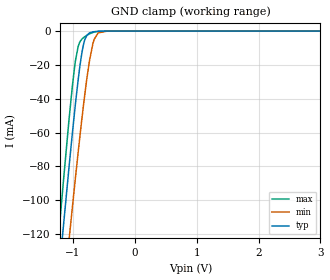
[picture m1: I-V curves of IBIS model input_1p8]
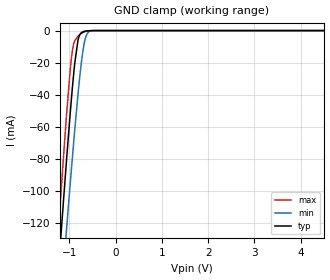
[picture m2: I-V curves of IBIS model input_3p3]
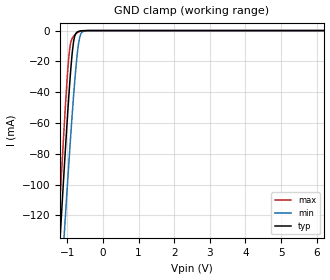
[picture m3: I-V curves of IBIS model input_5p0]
| Texas Instruments Incorporated
| ADS7028 Small, 8-Channel, 12-bit ADC with SPI Interface, GPIOs & CRC
[IBIS Ver]   4.1
[File name]   ads7028.ibs
[File Rev]   1.0
[Date]   03/21/2019
[Source]
| Texas Instruments Incorporated.
| Analog-eLab Design Center, HPA
| 12500 TI Blvd
| Dallas, TX -75243
[Notes]   Revision History:
| Rev 1.0: 03/21/2019
| - Initial version of the model
| - Model generated from simulations in SPECTRE
| - C_comp although listed in numerical order of value are
|   obtained from varying PVT conditions. For PVT conditions for
|   each specific value refer the buffer description under
|   respective [Model]. IBIS model user is responsible for using
|   appropriate C_comp to simulate for Signal Integrity.
| - Warnings regarding combined Non-monotonicity of various models have been
|   reviewd and considered minor and can be ignored.
| - Model names with a trailing _1p8 contain the model for 1.8V operation.
|   Model names with a trailing _2p5 contain the model for 2.5V operation.
|   Model names with a trailing _3p3 contain the model for 3.3V operation.
|   Model names with a trailing _5p0 contain the model for 5.0V operation.
[Disclaimer]
| This model is designed as an aid for customers of Texas Instruments.
| TI and its licensors and suppliers make no warranties, either expressed
| or implied, with respect to this  model, including the warranties of
| merchantability or fitness for a particular purpose. The model is
| provided solely on an "as is" basis. The entire risk as to its quality
| and performance is with the customer.
| This model is subject to change without notice. Texas Instruments
| Incorporated is not responsible for updating this model.
[Copyright]
 (C) Copyright 2019 Texas Instruments Incorporated.All rights reserved.
|  Component ADS7028RTE 16-Pin WQFN - RTE package
|  Part # ADS7028RTE
[Component]   ADS7028RTE
[Manufacturer]   TI
[Package]   |16 WQFN - RTE package
|   typ   min   max
R_pkg   0.05   0.04   0.06
L_pkg   1.0nH   0.8nH   1.2nH
C_pkg   0.2pF   0.16pF   0.24pF
[Pin]   signal_name   model_name   R_pin   L_pin   C_pin
1   AIN2/GPIO2   io   NA   NA   NA
2   AIN3/GPIO3   io   NA   NA   NA
3   AIN4/GPIO4   io   NA   NA   NA
4   AIN5/GPIO5   io   NA   NA   NA
5   AIN6/GPIO6   io   NA   NA   NA
6   AIN7/GPIO7   io   NA   NA   NA
7   AVDD   power   NA   NA   NA
8   DECAP   power   NA   NA   NA
9   GND   gnd   NA   NA   NA
10   DVDD   power   NA   NA   NA
11   CSb   input   NA   NA   NA
12   SDO   output   NA   NA   NA
13   SCLK   input   NA   NA   NA
14   SDI   input   NA   NA   NA
15   AIN0/GPIO0   io   NA   NA   NA
16   AIN1/GPIO1   io   NA   NA   NA
|   Model Selectors
[Model Selector] input
input_1p8   1.8V   digital input
input_3p3   3.3V   digital input
input_5p0   5.0V   digital input
[Model Selector] output
output_1p8   1.8V   digital output
output_3p3   3.3V   digital output
output_5p0   5.0V   digital output
[Model Selector] io
io_2p5   2.5V   digital I/O
io_3p3   3.3V   digital I/O
io_5p0   5.0V   digital I/O
| Models and submodels in the file (9): input_1p8 (Input), input_3p3 (Input), input_5p0 (Input), output_1p8 (3-state), output_3p3 (3-state), output_5p0 (3-state), io_2p5 (I/O), io_3p3 (I/O), io_5p0 (I/O)
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|   input_1p8 Model
[Model]   input_1p8
Model_type   Input
Vinl = 0.54
Vinh = 1.26
|   typ   min   max
C_comp   0.866pF   0.866pF   0.870pF
[Model spec]
|subparameter
Vinl   0.54   0.495   0.585
Vinh   1.26   1.155   1.365
| Where Nom  PVT is Nominal Process, 1.8V, 27C
|   Fast PVT is Strong Process,  1.95V, -40C
|   Slow PVT is Weak Process,   1.65V, 125C
[Voltage Range]   1.8   1.65   1.95
|Junction Temperature
[Temperature Range]   27   125   -40
[Power Clamp Reference]   1.8   1.65   1.95
[GND Clamp Reference]   0   0   0
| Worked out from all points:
|   GND clamp passes 1 mA (typ) near -0.72 V on its own axis
[GND Clamp]
|   Voltage   I(typ)   I(min)   I(max)
-1.8V     -381.3mA   -405mA     -375.1mA
-1.211V   -138.8mA   -179mA     -113.7mA
-1.157V   -117.4mA   -158.8mA   -90.96mA
-1.06V    -79.93mA   -123.2mA   -51.79mA
-957.6mV  -42.91mA   -86.69mA   -17.51mA
-914.4mV  -28.96mA   -71.87mA   -9.151mA
-849.6mV  -11.97mA   -50.62mA   -4.589mA
-806.4mV  -5.103mA   -37.41mA   -3.277mA
-730.8mV  -1.109mA   -17.52mA   -1.624mA
-655.2mV  -339.6uA   -4.922mA   -609uA
-444.6mV  -4.062uA   -21.46uA   -5.941uA
3.6V      0A         0A         0A
[POWER Clamp]
|   Voltage   I(typ)   I(min)   I(max)
-1.8V     0A         0A         0A
0V        0A         0A         0A
3.6V      0A         0A         0A
|   input_3p3 Model
[Model]   input_3p3
Model_type   Input
Vinl = 0.99
Vinh = 2.31
|   typ   min   max
C_comp   0.786pF   0.783pF   0.786pF
[Model spec]
|subparameter
Vinl   0.99   0.9   1.08
Vinh   2.31   2.1   2.52
| Where Nom  PVT is Nominal Process, 3.3V, 27C
|   Fast PVT is Strong Process,  3.6V, -40C
|   Slow PVT is Weak Process,   3.0V, 125C
[Voltage Range]   3.3   3   3.6
|Junction Temperature
[Temperature Range]   27   125   -40
[Power Clamp Reference]   3.3   3   3.6
[GND Clamp Reference]   0   0   0
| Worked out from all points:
|   GND clamp passes 1 mA (typ) near -0.72 V on its own axis
[GND Clamp]
|   Voltage   I(typ)   I(min)   I(max)
-3.3V     -1.017A    -997.3mA   -1.061A
-1.32V    -182.6mA   -219.9mA   -160.7mA
-1.211V   -138.7mA   -178.9mA   -113.6mA
-1.191V   -130.8mA   -171.5mA   -105.2mA
-1.063V   -80.84mA   -124mA     -52.71mA
-983.4mV  -51.83mA   -95.71mA   -24.76mA
-933.9mV  -35.08mA   -78.51mA   -12.26mA
-815.1mV  -6.145mA   -39.99mA   -3.51mA
-706.2mV  -740.5uA   -12.42mA   -1.222mA
-617.1mV  -188uA     -2.054mA   -330.8uA
-478.5mV  -10.73uA   -53.92uA   -17.39uA
6.6V      0A         0A         0A
[POWER Clamp]
|   Voltage   I(typ)   I(min)   I(max)
-3.3V     0A         0A         0A
0V        0A         0A         0A
6.6V      0A         0A         0A
|   input_5p0 Model
[Model]   input_5p0
Model_type   Input
Vinl = 1.5
Vinh = 3.5
|   typ   min   max
C_comp   0.724pF   0.724pF   0.727pF
[Model spec]
|subparameter
Vinl   1.5   1.35   1.65
Vinh   3.5   3.15   3.85
| Where Nom  PVT is Nominal Process, 5.0V, 27C
|   Fast PVT is Strong Process,  5.5V, -40C
|   Slow PVT is Weak Process,   4.5V, 125C
[Voltage Range]   5   4.5   5.5
|Junction Temperature
[Temperature Range]   27   125   -40
[Power Clamp Reference]   5   4.5   5.5
[GND Clamp Reference]   0   0   0
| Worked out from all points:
|   GND clamp passes 1 mA (typ) near -0.72 V on its own axis
[GND Clamp]
|   Voltage   I(typ)   I(min)   I(max)
-5V       -1.745A    -1.676A    -1.844A
-1.25V    -154.3mA   -193.4mA   -130.3mA
-1.145V   -112.6mA   -154.3mA   -85.81mA
-1.1V     -95.1mA    -137.7mA   -67.43mA
-1.055V   -77.98mA   -121.3mA   -49.8mA
-950mV    -40.36mA   -84.05mA   -15.66mA
-905mV    -26.14mA   -68.71mA   -8.036mA
-830mV    -8.329mA   -44.51mA   -3.939mA
-695mV    -621.9uA   -10.4mA    -1.062mA
-605mV    -154.6uA   -1.521mA   -268.7uA
-440mV    -3.526uA   -18.92uA   -5.052uA
10V       0A         0A         0A
[POWER Clamp]
|   Voltage   I(typ)   I(min)   I(max)
-5V       0A         0A         0A
0V        0A         0A         0A
10V       0A         0A         0A
